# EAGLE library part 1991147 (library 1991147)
PCB terminal block, nominal current: 24 A, rated voltage (III/2): 400 V, nominal cross section: 2.5 mm?, Number of potentials: 7, Number of rows: 1, Number of positions per row: 7, product range: SPT 2,5/..-V, pitch: 5 mm, connection method: Push-in spring connection, mounting: Wave soldering, conductor/PCB connection direction: 90 ?, color: green, Pin layout: Linear double pinning, Solder pin [P]: 2.5 mm, type of packaging: packed in cardboard Source: Datasheet
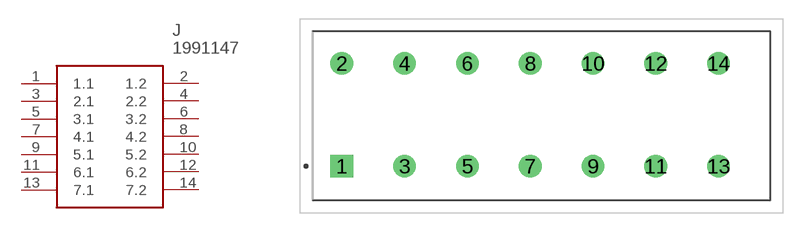
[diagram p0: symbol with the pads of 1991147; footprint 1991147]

Designator prefix J

## 1991147 (Description: PCB terminal block, nominal current: 24 A, rated voltage (III/2): 400 V, nominal cross section: 2.5 mm?, Number of potentials: 7, Number of rows: 1, Number of positions per row: 7, product range: SPT 2,5/..-V, pitch: 5 mm, connection method: Push-in spring connection, mounting: Wave soldering, conductor/PCB connection direction: 90 ?, color: green, Pin layout: Linear double pinning, Solder pin [P]: 2.5 mm, type of packaging: packed in cardboard; Height: 14.4mm; Manufacturer_Name: Phoenix Contact; Manufacturer_Part_Number: 1991147; Mouser_Part_Number: 651-1991147; Mouser_Price-Stock: https://www.mouser.com/Search/Refine.aspx?Keyword=651-1991147)  [1991147]
1  1.1
2  1.2
3  2.1
4  2.2
5  3.1
6  3.2
7  4.1
8  4.2
9  5.1
10  5.2
11  6.1
12  6.2
13  7.1
14  7.2

## Footprint 1991147 (pad centres in mm)
1991147
drill 1.2 pad 1.8 square: 1 0,0
drill 1.2 pad 1.8: 2 0,8.2; 3 5,0; 4 5,8.2; 5 10,0; 6 10,8.2; 7 15,0; 8 15,8.2; 9 20,0; 10 20,8.2; 11 25,0; 12 25,8.2; 13 30,0; 14 30,8.2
